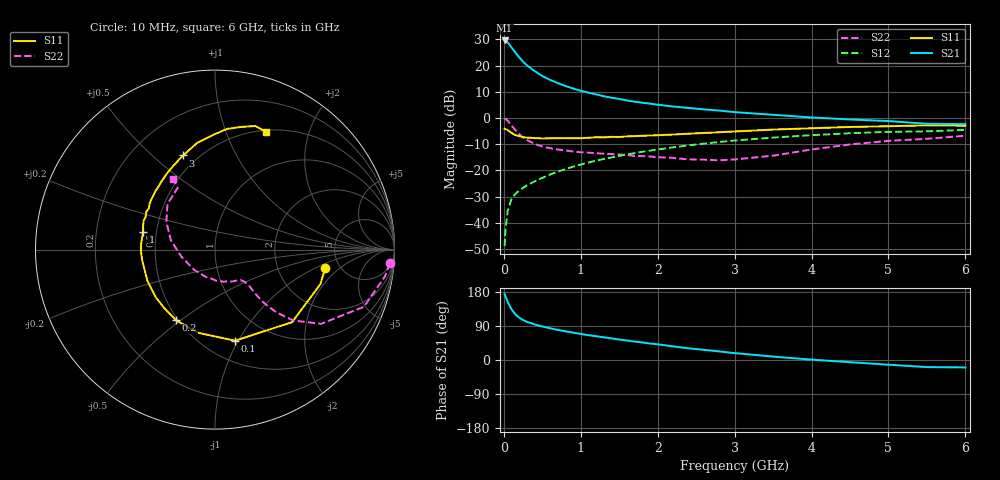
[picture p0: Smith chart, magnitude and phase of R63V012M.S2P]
! SIEMENS Small Signal Semiconductors
! BFR193
! Si NPN RF Bipolar Junction Transistor in SOT23
! VCE = 3 V  IC = 12 mA
! Common Emitter S-Parameters:  May  1996
# GHz  S  MA  R  50
!  f  S11  S21  S12  S22
! GHz  MAG  ANG  MAG  ANG  MAG  ANG  MAG  ANG
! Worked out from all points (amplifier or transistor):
!   36 points, 10 MHz to 6 GHz, reference 50 ohm
!   highest |S21| = 29.6 dB at 10 MHz (marker M1)
!   |S21| within 3 dB of that: start of sweep to 108.9 MHz
!   unconditionally stable (mu >= 1): 698.3 MHz to 2.014 GHz
!   at 250 MHz: K = 0.70, MSG = 24.0 dB, |S12| = -26.6 dB
!   at 1.4 GHz: K = 1.03, MAG = 10.3 dB, |S12| = -15.0 dB
!   at 6 GHz: K = 0.95, MSG = 1.1 dB, |S12| = -4.5 dB
!   S11 on the Smith chart (normalised r, x): 10 MHz: 3.86, -1.27; 100 MHz: 0.70, -0.97; 200 MHz: 0.49, -0.48; 1 GHz: 0.42, +0.10; 3 GHz: 0.42, +0.63; 6 GHz: 0.52, +1.39
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0.01  0.6228 -9.3  30.15 174.3  0.0036 85.4  0.9766 -4.5
0.02  0.6179 -18.1  29.67 168.4  0.0069 80.7  0.9585 -9.0
0.05  0.59 -43.2  27.68 153.1  0.0171 72.1  0.889 -21.0
0.1  0.5197 -77.6  22.26 133.6  0.0287 62.9  0.7211 -35.0
0.15  0.473 -101.4  17.57 120.3  0.0359 58.2  0.5876 -42.2
0.2  0.4496 -118.8  14.34 111.8  0.0411 57.0  0.4928 -45.5
0.25  0.4312 -130.9  11.87 105.4  0.0468 57.4  0.4255 -47.1
0.3  0.4239 -140.8  10.17 100.8  0.0518 58.1  0.3829 -47.6
0.4  0.4149 -155.0  7.851 94.0  0.0618 60.5  0.3214 -47.5
0.5  0.408 -164.5  6.346 88.4  0.0724 62.5  0.286 -46.8
0.6  0.4104 -172.0  5.345 83.7  0.0836 63.4  0.266 -46.7
0.8  0.4131 176.2  4.088 75.8  0.1061 64.1  0.2411 -47.7
1  0.4129 166.2  3.309 68.7  0.1297 64.4  0.2225 -49.9
1.1  0.421 162.3  3.051 65.5  0.1416 63.8  0.2186 -52.3
1.3  0.4277 154.7  2.602 59.8  0.1656 62.7  0.2087 -55.9
1.6  0.4462 144.6  2.157 51.4  0.2015 60.4  0.197 -64.5
2.2  0.4842 127.7  1.66 35.9  0.276 53.8  0.1738 -87.3
3  0.5539 108.7  1.295 18.2  0.372 42.6  0.1622 -135.6
3.5  0.6022 99.6  1.152 9.0  0.4237 35.0  0.1913 -168.3
4.5  0.6759 84.3  0.94 -5.8  0.5131 20.2  0.3131 150.0
5.5  0.7247 71.9  0.776 -18.7  0.5575 5.1  0.4017 121.1
6  0.7146 66.6  0.765 -19.6  0.5948 0.6  0.4595 120.8
